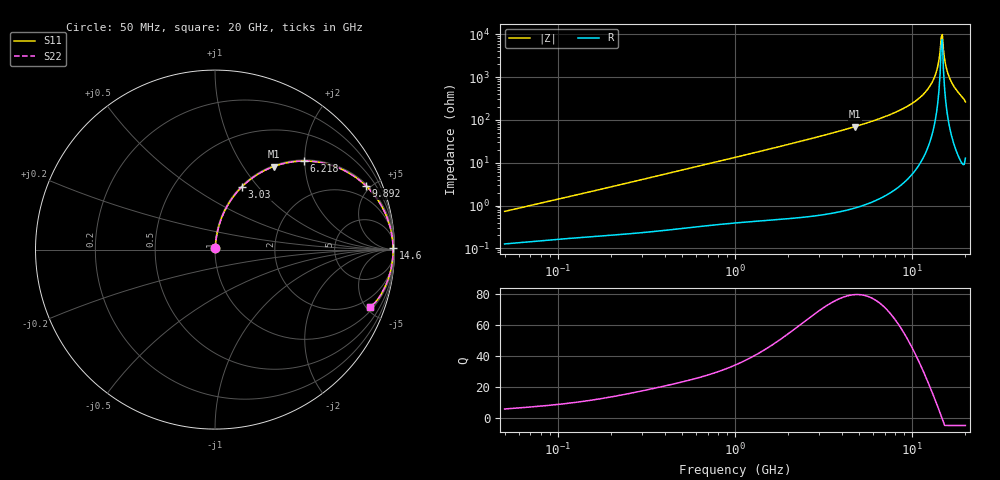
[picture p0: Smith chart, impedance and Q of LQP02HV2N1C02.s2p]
!Murata Part Number: LQP02HV2N1C02
!These Parameters are Measured in Series Mode Connection
!  o--[Z]--o
!Port1  Port2
!  o-------o
!Freq. Start=50[MHz] Stop=20[GHz], 401[Steps]
# Hz S RI R 50
!Freq.(Hz) S11(Real) S11(Imag) S21(Real) S21(Imag) S12(Real) S12(Imag) S22(Real) S22(Imag)
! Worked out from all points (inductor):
!   401 points, 50 MHz to 20 GHz, reference 50 ohm
!   read as one part in series: L = 2.26 nH near 51.52 MHz
!   highest Q = 79.6 at 4.748 GHz (marker M1), where L = 2.33 nH
!   self-resonance near 14.6 GHz
!   S11 on the Smith chart (normalised r, x): 50 MHz: 1.00, +0.01; 3.03 GHz: 1.01, +0.83; 6.218 GHz: 1.03, +1.98; 9.892 GHz: 1.10, +4.71; 14.6 GHz: open; 20 GHz: 1.26, -5.25
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5e7  0.00132 0.00715  0.9987 -0.00715  0.9987 -0.00715  0.00132 0.00715
1.364002e8  0.00215 0.0187  0.9979 -0.0187  0.9979 -0.0187  0.00215 0.0187
3.721004e8  0.00502 0.0497  0.995 -0.0497  0.995 -0.0497  0.00502 0.0497
1e9  0.021 0.1295  0.979 -0.1295  0.979 -0.1295  0.021 0.1295
2.728004e9  0.1244 0.3225  0.8756 -0.3225  0.8756 -0.3225  0.1244 0.3225
3.029571e9  0.1503 0.3503  0.8497 -0.3503  0.8497 -0.3503  0.1503 0.3503
4.748272e9  0.3271 0.4629  0.6729 -0.4629  0.6729 -0.4629  0.3271 0.4629
6.217679e9  0.4952 0.4934  0.5048 -0.4934  0.5048 -0.4934  0.4952 0.4934
7.442007e9  0.6291 0.4758  0.3709 -0.4758  0.3709 -0.4758  0.6291 0.4758
9.892087e9  0.8419 0.3542  0.1581 -0.3542  0.1581 -0.3542  0.8419 0.3542
1.166392e10  0.9364 0.2274  0.0636 -0.2274  0.0636 -0.2274  0.9364 0.2274
1.295331e10  0.9748 0.1297  0.0252 -0.1297  0.0252 -0.1297  0.9748 0.1297
1.375312e10  0.9872 0.0701  0.0128 -0.0701  0.0128 -0.0701  0.9872 0.0701
1.396067e10  0.9892 0.0549  0.0108 -0.0549  0.0108 -0.0549  0.9892 0.0549
1.438523e10  0.9917 0.0243  0.00829 -0.0243  0.00829 -0.0243  0.9917 0.0243
1.460232e10  0.9923 0.0089  0.00774 -0.0089  0.00774 -0.0089  0.9923 0.0089
1.482269e10  0.9923 -0.00649  0.00767 0.00649  0.00767 0.00649  0.9923 -0.00649
1.504638e10  0.9919 -0.0219  0.00808 0.0219  0.00808 0.0219  0.9919 -0.0219
1.573793e10  0.9878 -0.068  0.0122 0.068  0.0122 0.068  0.9878 -0.068
1.646126e10  0.9794 -0.1136  0.0206 0.1136  0.0206 0.1136  0.9794 -0.1136
1.774144e10  0.9558 -0.1876  0.0442 0.1876  0.0442 0.1876  0.9558 -0.1876
2e10  0.8616 -0.3218  0.1384 0.3218  0.1384 0.3218  0.8616 -0.3218
